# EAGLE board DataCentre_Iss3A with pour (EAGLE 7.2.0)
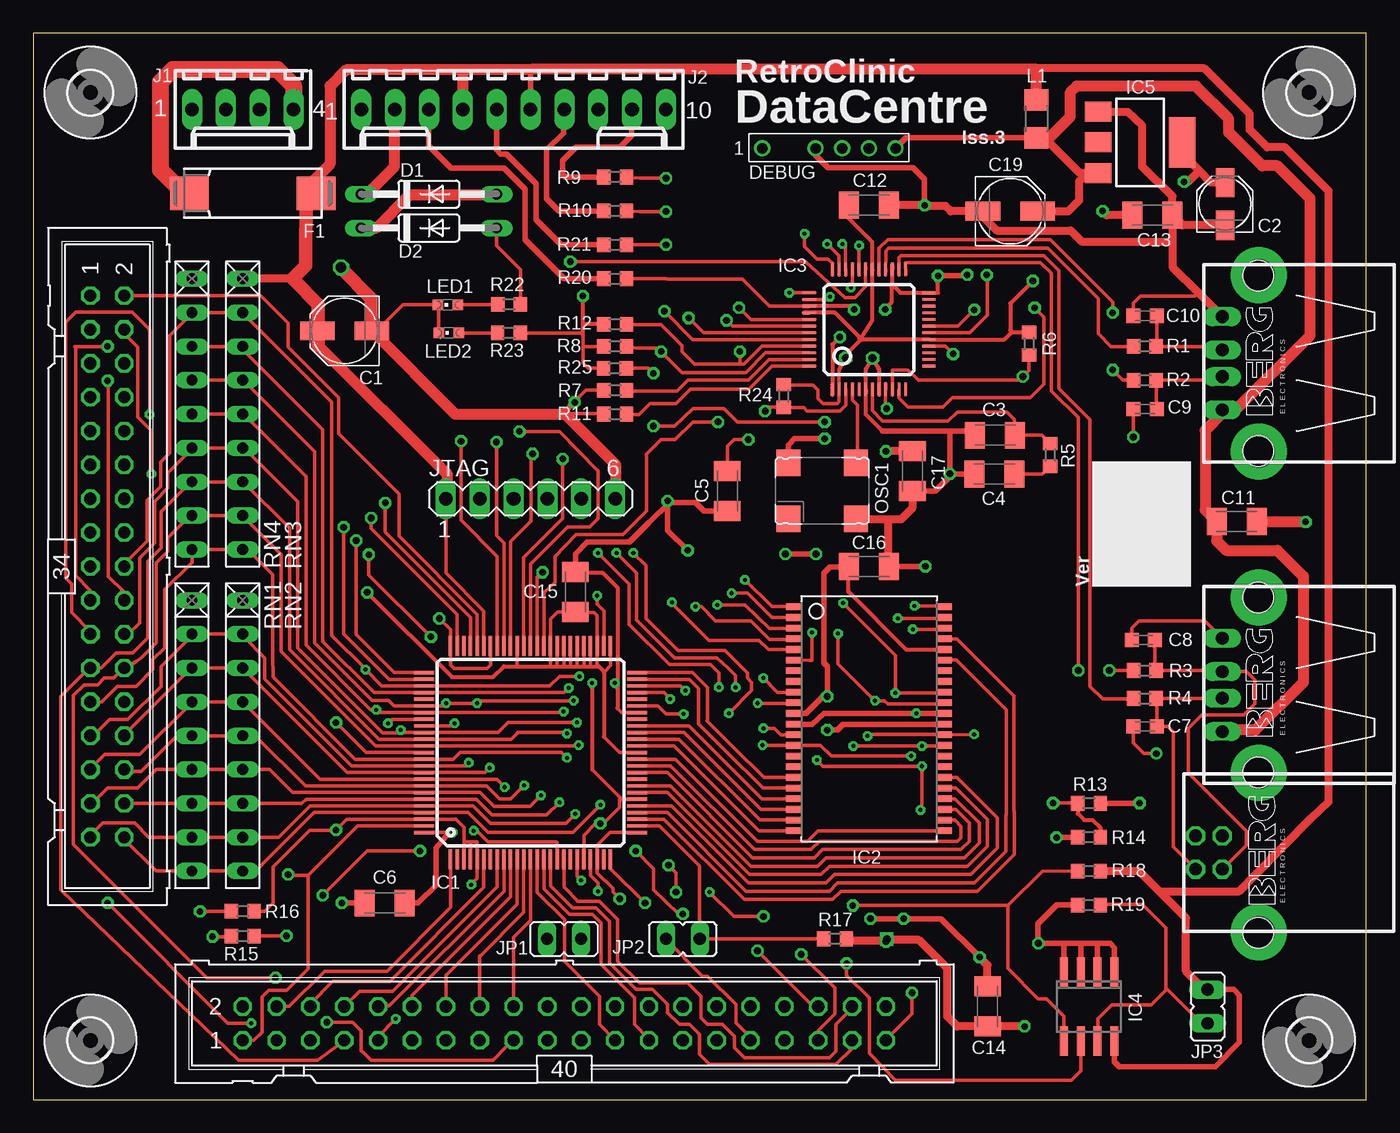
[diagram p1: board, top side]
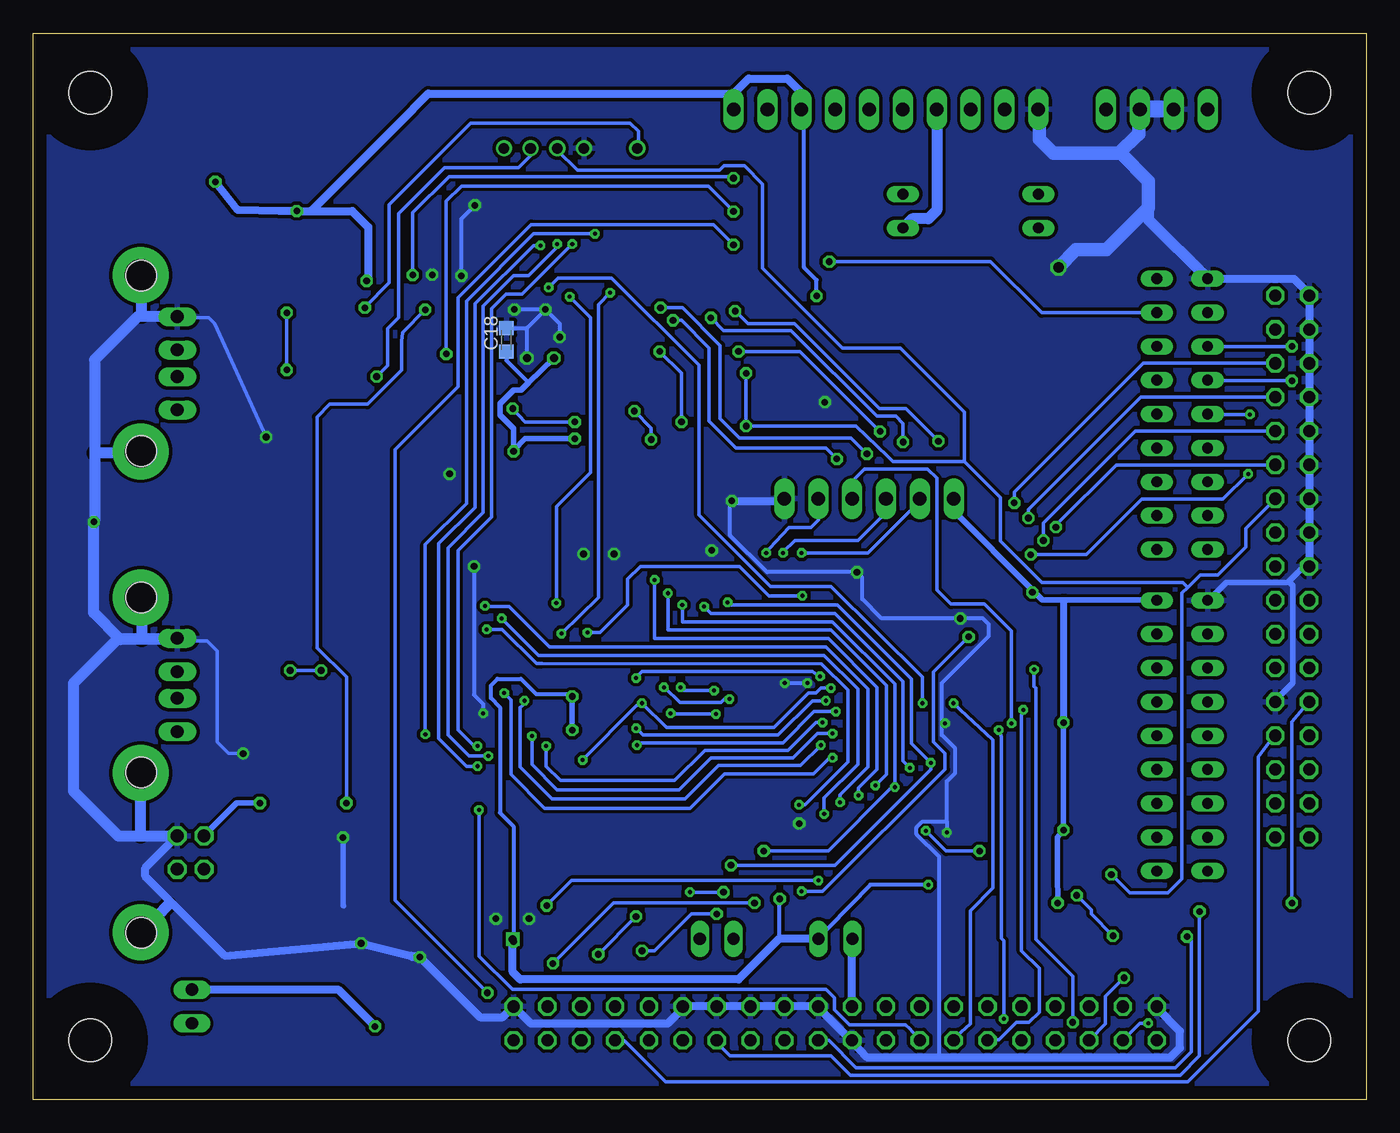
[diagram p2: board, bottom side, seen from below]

Size 100 x 80 mm. Coordinates in mm from the lower left corner, seen from the top.
Outline: 0,0 100,0 100,80 0,80 0,0
Copper layers (1*16): Top 0.035mm / dielectric 1.5mm / Bottom 0.035mm
Design rules "pcb-pool *": minimum track width 6mil, minimum drill 12mil, track to track 6mil, track to pad 6mil, pad to pad 6mil, via to via 6mil, smd to smd 8mil, copper to edge 40mil, drill to drill 20mil, minimum pad ring 8mil, minimum via ring 8mil, stop-mask expansion 3mil, vias tented up to drill 0mil, thermal gap 10mil
Net classes: 0 Signal: width 0.254 mm; 1 Power: width 0.305 mm

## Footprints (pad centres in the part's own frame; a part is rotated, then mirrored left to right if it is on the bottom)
PANASONIC_C = smd 2.6 x 1.4: + 2.05,0; - -2.05,0
PANASONIC_B = smd 2.2 x 1.4: + 1.6,0; - -1.6,0
C1206K = smd 1.5 x 2: 1 -1.5,0; 2 1.5,0
C0603K = smd 1.05 x 1.08: 1 -0.875,0; 2 0.875,0
DO35-10 = drill 0.813 long: A 5.08,0; C -5.08,0
DF3P-06 = drill 0.8: 1 -5,1; 3 -1,1; 4 1,1; 5 3,1; 6 5,1
085CS_1R = smd 2.9 x 2.5: + 4.75,0; - -4.75,0
TQ100 = smd 1.5 x 0.254: 1 -8,6; 2 -8,5.5; 3 -8,5; 4 -8,4.5; 5 -8,4; 6 -8,3.5; 7 -8,3; 8 -8,2.5; 9 -8,2; 10 -8,1.5; 11 -8,1; 12 -8,0.5; 13 -8,0; 14 -8,-0.5; 15 -8,-1; 16 -8,-1.5; 17 -8,-2; 18 -8,-2.5; 19 -8,-3; 20 -8,-3.5; 21 -8,-4; 22 -8,-4.5; 23 -8,-5; 24 -8,-5.5; 25 -8,-6; 51 8,-6; 52 8,-5.5; 53 8,-5; 54 8,-4.5; 55 8,-4; 56 8,-3.5; 57 8,-3; 58 8,-2.5; 59 8,-2; 60 8,-1.5; 61 8,-1; 62 8,-0.5; 63 8,0; 64 8,0.5; 65 8,1; 66 8,1.5; 67 8,2; 68 8,2.5; 69 8,3; 70 8,3.5; 71 8,4; 72 8,4.5; 73 8,5; 74 8,5.5; 75 8,6 | smd 0.254 x 1.5: 26 -6,-8; 27 -5.5,-8; 28 -5,-8; 29 -4.5,-8; 30 -4,-8; 31 -3.5,-8; 32 -3,-8; 33 -2.5,-8; 34 -2,-8; 35 -1.5,-8; 36 -1,-8; 37 -0.5,-8; 38 0,-8; 39 0.5,-8; 40 1,-8; 41 1.5,-8; 42 2,-8; 43 2.5,-8; 44 3,-8; 45 3.5,-8; 46 4,-8; 47 4.5,-8; 48 5,-8; 49 5.5,-8; 50 6,-8; 76 6,8; 77 5.5,8; 78 5,8; 79 4.5,8; 80 4,8; 81 3.5,8; 82 3,8; 83 2.5,8; 84 2,8; 85 1.5,8; 86 1,8; 87 0.5,8; 88 0,8; 89 -0.5,8; 90 -1,8; 91 -1.5,8; 92 -2,8; 93 -2.5,8; 94 -3,8; 95 -3.5,8; 96 -4,8; 97 -4.5,8; 98 -5,8; 99 -5.5,8; 100 -6,8
TSOPII-Z44 = smd 0.5 x 1.2: 1 -8.4,-5.627; 2 -7.6,-5.627; 3 -6.8,-5.627; 4 -6,-5.627; 5 -5.2,-5.627; 6 -4.4,-5.627; 7 -3.6,-5.627; 8 -2.8,-5.627; 9 -2,-5.627; 10 -1.2,-5.627; 11 -0.4,-5.627; 12 0.4,-5.627; 13 1.2,-5.627; 14 2,-5.627; 15 2.8,-5.627; 16 3.6,-5.627; 17 4.4,-5.627; 18 5.2,-5.627; 19 6,-5.627; 20 6.8,-5.627; 21 7.6,-5.627; 22 8.4,-5.627; 23 8.4,5.627; 24 7.6,5.627; 25 6.8,5.627; 26 6,5.627; 27 5.2,5.627; 28 4.4,5.627; 29 3.6,5.627; 30 2.8,5.627; 31 2,5.627; 32 1.2,5.627; 33 0.4,5.627; 34 -0.4,5.627; 35 -1.2,5.627; 36 -2,5.627; 37 -2.8,5.627; 38 -3.6,5.627; 39 -4.4,5.627; 40 -5.2,5.627; 41 -6,5.627; 42 -6.8,5.627; 43 -7.6,5.627; 44 -8.4,5.627
LQFP48 = smd 0.2 x 1: 1 -2.75,-4.5; 2 -2.25,-4.5; 3 -1.75,-4.5; 4 -1.25,-4.5; 5 -0.75,-4.5; 6 -0.25,-4.5; 7 0.25,-4.5; 8 0.75,-4.5; 9 1.25,-4.5; 10 1.75,-4.5; 11 2.25,-4.5; 12 2.75,-4.5; 25 2.75,4.5; 26 2.25,4.5; 27 1.75,4.5; 28 1.25,4.5; 29 0.75,4.5; 30 0.25,4.5; 31 -0.25,4.5; 32 -0.75,4.5; 33 -1.25,4.5; 34 -1.75,4.5; 35 -2.25,4.5; 36 -2.75,4.5 | smd 1 x 0.2: 13 4.5,-2.75; 14 4.5,-2.25; 15 4.5,-1.75; 16 4.5,-1.25; 17 4.5,-0.75; 18 4.5,-0.25; 19 4.5,0.25; 20 4.5,0.75; 21 4.5,1.25; 22 4.5,1.75; 23 4.5,2.25; 24 4.5,2.75; 37 -4.5,2.75; 38 -4.5,2.25; 39 -4.5,1.75; 40 -4.5,1.25; 41 -4.5,0.75; 42 -4.5,0.25; 43 -4.5,-0.25; 44 -4.5,-0.75; 45 -4.5,-1.25; 46 -4.5,-1.75; 47 -4.5,-2.25; 48 -4.5,-2.75
SO-08 = smd 0.6 x 2.2: 1 -1.905,-2.6; 2 -0.635,-2.6; 3 0.635,-2.6; 4 1.905,-2.6; 5 1.905,2.6; 6 0.635,2.6; 7 -0.635,2.6; 8 -1.905,2.6
SOT223 = smd 1.5 x 2: 1 -2.3,-3.15; 2 0,-3.15; 3 2.3,-3.15 | smd 3.8 x 2: 4 0,3.15
ML40 = drill 0.914 octagon: 1 -24.13,-1.27; 2 -24.13,1.27; 3 -21.59,-1.27; 4 -21.59,1.27; 5 -19.05,-1.27; 6 -19.05,1.27; 7 -16.51,-1.27; 8 -16.51,1.27; 9 -13.97,-1.27; 10 -13.97,1.27; 11 -11.43,-1.27; 12 -11.43,1.27; 13 -8.89,-1.27; 14 -8.89,1.27; 15 -6.35,-1.27; 16 -6.35,1.27; 17 -3.81,-1.27; 18 -3.81,1.27; 19 -1.27,-1.27; 20 -1.27,1.27; 21 1.27,-1.27; 22 1.27,1.27; 23 3.81,-1.27; 24 3.81,1.27; 25 6.35,-1.27; 26 6.35,1.27; 27 8.89,-1.27; 28 8.89,1.27; 29 11.43,-1.27; 30 11.43,1.27; 31 13.97,-1.27; 32 13.97,1.27; 33 16.51,-1.27; 34 16.51,1.27; 35 19.05,-1.27; 36 19.05,1.27; 37 21.59,-1.27; 38 21.59,1.27; 39 24.13,-1.27; 40 24.13,1.27
6410-04 = drill 1.016 long: 1 3.81,0; 2 1.27,0; 3 -1.27,0; 4 -3.81,0
6410-10 = drill 1.016 long: 1 11.43,0; 2 8.89,0; 3 6.35,0; 4 3.81,0; 5 1.27,0; 6 -1.27,0; 7 -3.81,0; 8 -6.35,0; 9 -8.89,0; 10 -11.43,0
JP1 = drill 0.914 long: 1 0,-1.27; 2 0,1.27
MA06-1 = drill 1.016 long: 1 -6.35,0; 2 -3.81,0; 3 -1.27,0; 4 1.27,0; 5 3.81,0; 6 6.35,0
R1206 = smd 1.6 x 1.803: 1 -1.422,0; 2 1.422,0
CHIPLED_0603 = smd 0.8 x 0.8: A 0,-0.75; C 0,0.75
XTAL-CSX750 = smd 1.8 x 2: 1 -2.54,-2.1; 2 2.54,-2.1; 3 2.54,2.1; 4 -2.54,2.1
ML34 = drill 0.914 octagon: 1 -20.32,-1.27; 2 -20.32,1.27; 3 -17.78,-1.27; 4 -17.78,1.27; 5 -15.24,-1.27; 6 -15.24,1.27; 7 -12.7,-1.27; 8 -12.7,1.27; 9 -10.16,-1.27; 10 -10.16,1.27; 11 -7.62,-1.27; 12 -7.62,1.27; 13 -5.08,-1.27; 14 -5.08,1.27; 15 -2.54,-1.27; 16 -2.54,1.27; 17 0,-1.27; 18 0,1.27; 19 2.54,-1.27; 20 2.54,1.27; 21 5.08,-1.27; 22 5.08,1.27; 23 7.62,-1.27; 24 7.62,1.27; 25 10.16,-1.27; 26 10.16,1.27; 27 12.7,-1.27; 28 12.7,1.27; 29 15.24,-1.27; 30 15.24,1.27; 31 17.78,-1.27; 32 17.78,1.27; 33 20.32,-1.27; 34 20.32,1.27
R0603 = smd 1 x 1.1: 1 -0.85,0; 2 0.85,0
RN-9 = drill 0.813 long: 1 -10.16,0; 2 -7.62,0; 3 -5.08,0; 4 -2.54,0; 5 0,0; 6 2.54,0; 7 5.08,0; 8 7.62,0; 9 10.16,0
3,2 = hole 3.2: 0,0
PN87520 = drill 0.95 long: 1 -3.5,2.71; 2 -1,2.71; 3 1,2.71; 4 3.5,2.71 | hole 2.3: -6.57,0; 6.57,0
PN61729 = drill 0.95 octagon: 1 1.25,4.71; 2 -1.25,4.71; 3 -1.25,2.71; 4 1.25,2.71 | hole 2.3: -6.02,0; 6.02,0

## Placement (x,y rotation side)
C1  47uF  [PANASONIC_C]  23.36,57.68 180 top
C2  22uF  [PANASONIC_B]  89.4,67.19 90 top
C3  1nF  [C1206K]  72.16,49.85 0 top
C4  10nF  [C1206K]  72.1,46.94 180 top
C5  100nF  [C1206K]  52.07,45.68 270 top
C6  100nF  [C1206K]  26.36,14.74 0 top
C7  47pF  [C0603K]  83.41,27.99 0 top
C8  47pF  [C0603K]  83.28,34.48 0 top
C9  47pF  [C0603K]  83.41,51.81 0 top
C10  47pF  [C0603K]  83.41,58.8 0 top
C11  100nF  [C1206K]  90.28,43.37 0 top
C12  100nF  [C1206K]  62.7,67.11 0 top
C13  100nF  [C1206K]  83.97,66.35 0 top
C14  100nF  [C1206K]  71.59,6.98 90 top
C15  100nF  [C1206K]  40.67,38.09 90 top
C16  100nF  [C1206K]  62.7,40 0 top
C17  100nF  [C1206K]  65.95,47.16 270 top
C18  100nF  [C0603K]  64.51,57.01 90 bottom
C19  47uF  [PANASONIC_C]  73.3,66.65 0 top
D1  1N4001  [DO35-10]  29.68,67.94 0 top
D2  1N4001  [DO35-10]  29.68,65.4 0 top
DEBUG  [DF3P-06]  59.69,70.37 0 top
F1  [085CS_1R]  16.47,68 180 top
IC1  XC9572TQ100  [TQ100]  37.3,26.03 90 top
IC2  62LV8001  [TSOPII-Z44]  62.7,28.57 270 top
IC3  VNC1L-1A  [LQFP48]  62.7,57.78 0 top
IC4  24LC512  [SO-08]  79.21,6.98 180 top
IC5  TS1117BCW33  [SOT223]  83.05,71.82 270 top
IDE  IDE  [ML40]  39.84,5.71 0 top
J1  22-27-2041-04  [6410-04]  15.71,74.29 180 top
J2  22-27-2101-10  [6410-10]  36.03,74.29 180 top
JP1  IDEPWR  [JP1]  39.82,12.06 90 top
JP2  SEL  [JP1]  48.73,12.06 90 top
JP3  WPROT  [JP1]  88.1,6.98 0 top
JTAG  [MA06-1]  37.3,45.08 0 top
L1  600R  [R1206]  75.25,73.58 90 top
LED1  [CHIPLED_0603]  31.11,59.63 90 top
LED2  [CHIPLED_0603]  31.17,57.52 90 top
OSC1  [XTAL-CSX750]  59.19,45.68 0 top
PL1  1MHZ  [ML34]  5.55,40 270 top
R1  27R  [R0603]  83.39,56.51 0 top
R2  27R  [R0603]  83.39,53.97 0 top
R3  27R  [R0603]  83.39,32.19 0 top
R4  27R  [R0603]  83.39,30.09 0 top
R5  180R  [R0603]  76.29,48.37 90 top
R6  47K  [R0603]  74.71,56.71 90 top
R7  47K  [R0603]  43.65,53.21 0 top
R8  47K  [R0603]  43.65,56.51 0 top
R9  330R  [R0603]  43.65,69.21 0 top
R10  330R  [R0603]  43.65,66.67 0 top
R11  10K  [R0603]  43.65,51.43 180 top
R12  47K  [R0603]  43.65,58.17 180 top
R13  100K  [R0603]  79.21,22.22 0 top
R14  100K  [R0603]  79.21,19.68 0 top
R15  1k  [R0603]  15.72,12.26 180 top
R16  4k7  [R0603]  15.72,14.13 180 top
R17  4k7  [R0603]  60.16,12.06 0 top
R18  4k7  [R0603]  79.21,17.14 0 top
R19  4k7  [R0603]  79.21,14.6 0 top
R20  470R  [R0603]  43.65,61.59 180 top
R21  470R  [R0603]  43.65,64.13 0 top
R22  470R  [R0603]  35.7,59.66 180 top
R23  330R  [R0603]  35.69,57.52 180 top
R24  0R  [R0603]  56.29,52.79 270 top
R25  47K  [R0603]  43.62,54.87 0 top
RN1  2k2  [RN-9]  11.9,27.3 270 top
RN2  2k2  [RN-9]  15.71,27.3 270 top
RN3  2k2  [RN-9]  15.71,51.43 270 top
RN4  2k2  [RN-9]  11.9,51.43 270 top
U$1  [3,2]  95.72,75.56 0 top
U$2  [3,2]  95.72,4.44 0 top
U$3  [3,2]  4.28,4.44 0 top
U$4  [3,2]  4.28,75.56 0 top
X1  USB2  [PN87520]  91.91,55.24 90 top
X2  USB1A  [PN87520]  91.91,31.11 90 top
X3  USB1B  [PN61729]  91.91,18.54 90 top

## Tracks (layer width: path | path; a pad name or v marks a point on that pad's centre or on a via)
!ACT  (via drill 0.5)
  Top 0.254: v65.93,8 65.93,6.43 63.97,4.47 IDE.39 | v47.47,64.13 R21.2
  Bottom 0.254: v65.93,8 72.86,14.93 72.86,48.76 68.13,53.49 68.13,60.16 62.65,65.65 48.98,65.65 48.97,65.63 v47.47,64.13
!DACK  (via drill 0.5)
  Top 0.254: 42.37,47.13 42.37,43.6 41.73,42.97 40.1,42.97 37.3,40.17 IC1.63 | 42.37,47.13 42.37,47.19 | IC3.46 54.92,56.03 53.45,54.56 48.66,54.56 47.03,56.19 | 47.03,56.19 46.84,56.39 45.27,56.39 R8.2 | v47.1,56.13 46.97,56.13 47.03,56.19 | v36.47,50.13 39.47,50.13 42.34,47.19 42.37,47.13
  Bottom 0.254: v47.1,56.13 42.47,56.13 v36.47,50.13
!DREQ  (via drill 0.5)
  Top 0: IC3.45 58.22,56.51 58.22,56.53
  Top 0.254: 58.64,56.53 58.22,56.53 54.67,56.53 53.33,55.19 53.14,55.19 | 58.64,56.53 IC3.45 | 53.14,55.19 49.61,55.19 48.66,56.13 48.66,56.57 47.09,58.15 44.52,58.15 R12.1 | v51.37,50.84 49.48,50.84 48.16,49.52 47.09,49.52 46.02,48.45 46.02,44.16 44.25,42.4 40.73,42.4 39.15,40.76 39.15,38.81 38.33,38.05 38.3,38.02 IC1.61 | v53.01,56.13 53.01,55.31 53.14,55.19
  Bottom 0.254: v51.37,50.84 51.37,54.5 v53.01,56.13
!IDECS0
  Top 0.254: IDE.37 61.41,3.81 60.22,2.63 50.72,2.63 49.97,3.38 49.97,4.88 49.22,5.63 48.47,5.63 47.59,6.5 47.59,7.13 46.47,8.26 45.22,8.26 43.22,10.26 43.22,13.38 42.22,14.38 40.47,14.38 38.8,16.05 IC1.16
!IDECS1
  Top 0.254: IDE.38 61.43,6.84 60.22,5.63 60.22,3.63 59.72,3.13 53.34,3.13 52.59,3.88 52.59,4.75 51.72,5.63 50.59,5.63 50.09,6.13 50.09,7.75 49.09,8.76 45.47,8.76 43.84,10.38 43.84,13.51 42.47,14.88 40.89,14.88 | 40.84,14.88 40.89,14.88 | IC1.18 39.8,15.97 40.89,14.88
!IDEINT
  Top 0.254: IDE.31 53.81,4.67 52.72,5.75 52.72,7.13 50.59,9.26 50.22,9.26 47.41,12.06 | 47.41,12.06 47.34,12.13 | 47.41,12.06 JP2.2
!IDEINTA
  Top 0.254: R17.1 JP2.1 49.98,12.08 49.98,17.52 46.97,20.53 IC1.27
!IDERD
  Top 0.254: IDE.25 46.19,4.54 45.09,5.63 45.09,7.63 42.59,10.13 42.59,13.26 41.97,13.88 40.22,13.88 38.3,15.8 IC1.15
!IDEWR
  Top 0.254: IDE.23 42.47,5.63 42.47,7.75 39.84,10.38 39.84,13.51 37.8,15.55 IC1.14
!IRQ  (via drill 0.5 pad 0.25)
  Top 0.254: 31.81,33.97 IC1.74 31.8,36.4 25.36,42.84 25.36,43.63 v25.34,43.64
  Bottom 0.254: PL1.8 16.9,52.7 25.34,44.26 v25.34,43.64
!NMI  (via drill 0.5 pad 0.25)
  Top 0.254: v26.41,44.76 26.41,42.57 32.8,36.18 IC1.72
  Bottom 0.254: PL1.6 16.73,55.24 26.41,45.57 v26.41,44.76
!PGFC  (via drill 0.5 pad 0.25)
  Top 0.254: v24.22,41.94 24.22,34.88 27.07,32.03 IC1.76
  Bottom 0.254: PL1.10 17.31,50.16 24.22,43.26 v24.22,41.94
!PGFD  (via drill 0.5 pad 0.25)
  Top 0.254: v23.28,42.94 23.28,34.94 26.7,31.53 IC1.77
  Bottom 0.254: PL1.12 18.73,47.62 23.28,43.09 23.28,42.82 v23.28,42.94
!RCE  (via drill 0.3)
  Top 0.254: v58.43,35.03 58.43,32.95 58.24,32.95 IC2.6 | v42.3,37.8 42.3,37.17 42.81,36.67 42.81,34.78 IC1.52
  Bottom 0.254: v58.43,35.03 57.48,35.03 55.41,37.11 55.41,39.06 54.46,40.01 47.03,40.01 44.82,37.8 v42.3,37.8
!ROE
  Top 0.254: IC2.41 69.28,34.57 73.55,30.29 73.55,21.67 73.59,21.63 73.59,18.38 70.84,15.63 60.59,15.63 59.97,15.01 53.34,15.01 47.32,21.03 IC1.28 45.24,21.03
!RST  (via drill 0.5)
  Top 0.254: IDE.1 16.53,4.43 17.16,5.06 17.16,7.7 17.67,8.19 18.99,8.19 20.6,9.8 20.6,16.81 | 29.32,20.53 IC1.99 24.32,20.53 20.6,16.81 | v64.04,51.85 63.95,51.96 63.95,53.72 IC3.9 | v46.52,50.53 48.1,50.53 49.48,51.85 51.81,51.85 52.82,50.84 v59.38,50.84 | R25.2 46.14,54.87 v46.52,54.5 | 20.6,16.81 19.19,16.81 v19.12,16.88
  Bottom 0.254: PL1.14 7.32,44.55 9.04,42.84 9.04,41.45 11.12,39.38 12.44,39.38 13.38,38.43 | 13.38,38.43 13.83,37.99 13.83,16.57 14.9,15.5 17.73,15.5 v19.12,16.88 | 30.14,47.88 35.5,47.88 35.88,48.26 38.27,50.53 v46.52,50.53 v46.52,54.5 | 30.14,47.88 27.43,45.17 27.43,41.9 24.35,38.81 13.76,38.81 13.38,38.43 | DEBUG.4 60.69,71.24 59.17,69.72 48.52,69.72 48.19,70.06 46.65,70.06 45.29,68.66 45.29,62.4 39.28,56.39 34.93,56.39 30.14,51.6 30.14,47.88 | v59.38,50.84 63.09,50.84 v64.04,51.85
!RWE
  Top 0.254: IC2.17 54.8,24.17 52.51,26.46 50.56,28.41 50.57,28.42 50.57,30.92 49.46,32.03 IC1.50 45.24,32.03
AD0  (via drill 0.3, 0.5)
  Top 0.254: RN1.2 11.88,34.92 11.85,34.88 | RN1.2 RN2.2 15.71,34.77 15.73,34.77 17.35,33.14 17.35,31.56 23.89,25.03 IC1.90 32.43,25.03 v32.66,25.26 | RN1.2 11.9,34.81 9.6,32.51 9.6,31 7.09,28.5 5.72,28.5 4.34,27.13 4.28,27.2 PL1.27 | v47.91,37.3 47.91,37.23 50.68,34.46 54.46,34.46 55.15,33.77 57.11,33.77 57.1,33.77 IC2.5 | v50.74,15.56 52.57,13.73 v54.78,13.73 | v47.66,17.58 48.22,17.01 v48.22,15.56 | IDE.35 58.87,5.17 60.13,6.43 60.13,8.38 v57.61,10.9
  Bottom 0.254: v47.91,37.3 47.72,37.11 39.66,37.11 34.11,31.56 34.11,26.71 v32.66,25.26 32.66,24.76 39.84,17.58 v47.66,17.58 | v48.22,15.56 v50.74,15.56 | v57.61,10.9 v54.78,13.73
AD1  (via drill 0.3)
  Top 0.254: RN2.3 | 11.9,32.45 11.85,32.51 | 11.9,32.45 RN1.3 11.85,32.38 6.82,27.36 PL1.28 | RN2.3 11.97,32.38 11.9,32.45 | v49.67,36.98 50.11,36.98 51.19,35.91 53.83,35.91 55.22,34.52 57.11,34.52 57.07,34.56 IC2.4 | RN2.3 23.56,24.53 IC1.91 33.88,24.53 v34.24,24.88
  Bottom 0.254: v34.24,24.88 34.74,25.39 34.74,31.37 39.84,36.48 49.17,36.48 v49.67,36.98 | IDE.33 55.97,4.41 55.66,4.41 52.57,1.32 13.38,1.32 8.09,6.62 8.09,25.7 7.34,26.71 PL1.28
AD2  (via drill 0.3, 0.5)
  Top 0.254: RN2.4 15.76,29.84 | RN1.4 11.68,29.84 11.6,29.75 | RN1.4 RN2.4 | RN1.4 11.9,29.81 7.97,25.88 5.34,25.88 4.28,24.81 PL1.29 | v51.31,37.11 53.39,37.11 55.22,35.34 57.17,35.34 57.14,35.37 IC2.3 | v54.34,11.15 58.24,7.25 IDE.36 | v45.2,18.65 46.52,17.32 46.52,15.75 48.41,13.92 v48.73,13.92 | v35.37,23.44 34.78,24.03 IC1.92 21.52,24.03 RN2.4
  Bottom 0.254: v51.31,37.11 51.31,35.85 40.03,35.85 35.37,31.18 v35.37,23.44 35.62,23.44 40.35,18.65 v45.2,18.65 | v54.34,11.15 53.39,11.15 50.62,13.92 v48.73,13.92
AD3  (via drill 0.3)
  Top 0.254: RN1.5 11.85,27.25 | RN1.5 RN2.5 15.75,27.26 16.7,27.26 20.43,23.53 IC1.93 34.02,23.53 35,22.55 35.81,22.55 v36.82,23.56 | RN1.5 10.77,27.3 8.1,24.63 6.97,24.63 6.84,24.76 PL1.30 | v52.38,37.99 53.58,37.99 55.41,36.16 57.04,36.16 57.05,36.17 IC2.2
  Bottom 0.254: v36.82,23.56 36,24.38 36,31.06 40.16,35.22 52.38,35.22 v52.38,37.99
AD4  (via drill 0.3)
  Top 0.254: RN1.6 11.73,24.76 11.72,24.75 | RN1.6 RN2.6 17.71,24.76 19.45,23.03 IC1.94 33.51,23.03 34.55,21.99 37.26,21.99 v38.08,22.81 | RN1.6 9.23,24.76 7.84,23.38 5.59,23.38 4.34,22.13 4.28,22.2 PL1.31 | v53.39,39 55.41,36.98 57.04,36.98 57.05,36.97 IC2.1
  Bottom 0.254: v38.08,22.81 38.08,23.37 36.7,24.76 36.7,30.93 40.35,34.59 53.39,34.59 v53.39,39
AD5  (via drill 0.3)
  Top 0.254: 15.71,22.24 15.72,22.25 | 15.71,22.24 RN2.7 20.14,22.22 20.45,22.53 IC1.95 33.25,22.53 34.43,21.36 38.52,21.36 v39.47,22.3 | 15.71,22.24 15.69,22.22 RN1.7 PL1.32 6.75,22.22 6.72,22.25 | IC2.44 68.33,36.99 68.38,37.04 v66.12,37.04
  Bottom 0.254: v39.47,22.3 39.47,22.87 37.39,24.95 37.39,30.81 40.54,33.96 61.27,33.96 64.29,36.98 66.05,36.98 v66.12,37.04
AD6  (via drill 0.3)
  Top 0.254: RN1.8 11.77,19.68 11.72,19.63 | RN1.8 RN2.8 18.42,19.68 20.77,22.03 IC1.96 33,22.03 34.3,20.73 39.97,20.73 v40.66,21.42 | RN1.8 8.67,19.68 7.59,20.75 5.22,20.75 4.22,19.75 4.28,19.7 PL1.33 | IC2.43 68.33,36.22 68.32,36.23 68.19,36.1 v64.86,36.1
  Bottom 0.254: v40.66,21.42 40.66,22.62 38.14,25.14 38.14,30.81 40.66,33.33 62.08,33.33 v64.86,36.1
AD7  (via drill 0.3)
  Top 0.254: 29.32,21.53 IC1.97 | 11.97,17.14 RN1.9 9.21,17.14 6.72,19.63 6.77,19.68 PL1.34 | 11.97,17.14 RN2.9 16.69,17.14 21.08,21.53 IC1.97 | 11.97,17.14 11.97,17 | v42.55,22.11 40.48,20.03 34.11,20.03 32.62,21.53 IC1.97 | IC2.42 68.36,35.37 68.38,35.34 68.32,35.28 v65.99,35.28
  Bottom 0.254: v42.55,22.11 42.11,22.11 38.9,25.33 38.9,30.74 40.85,32.7 61.82,32.73 | 61.82,32.73 61.91,32.73 | v65.99,35.28 64.83,35.28 62.23,32.73 61.87,32.73 61.82,32.73
ADR8
  Top 0.254: IC2.39 69.25,32.97 72.99,29.23 72.99,21.36 72.97,21.38 72.97,18.63 70.59,16.25 60.34,16.25 59.72,15.63 53.47,15.63 47.57,21.53 IC1.29
ADR9
  Top 0.254: IC2.28 69.3,24.17 72.34,21.13 72.34,18.88 70.34,16.88 60.09,16.88 59.47,16.25 53.65,16.25 47.88,22.03 IC1.30
ADR10
  Top 0.254: IC2.27 69.23,23.37 71.59,21 71.59,19 70.09,17.5 59.72,17.5 59.09,16.88 53.72,16.88 47.57,23.03 IC1.32
ADR11
  Top 0.254: IC2.26 69.16,22.57 70.97,20.75 70.97,19.25 69.84,18.13 59.47,18.13 58.84,17.5 53.84,17.5 47.82,23.53 IC1.33
ADR12
  Top 0.254: IC2.25 69.2,21.77 70.22,20.75 70.22,19.38 69.59,18.75 59.22,18.75 58.59,18.13 53.97,18.13 47.57,24.53 IC1.35
ADR13
  Top 0.254: IC2.24 69.13,20.97 69.59,20.5 69.59,19.63 69.34,19.38 58.97,19.38 58.34,18.75 54.09,18.75 47.82,25.03 IC1.36 45.24,25.03
ADR14
  Top 0.254: IC2.23 58.88,20.17 58.09,19.38 54.34,19.38 48.2,25.53 IC1.37
ADR15
  Top 0.254: IC2.22 54.43,20.17 48.07,26.53 IC1.39
ADR16
  Top 0.254: IC2.21 54.5,20.97 48.45,27.03 IC1.40 45.24,27.03
ADR17
  Top 0.254: IC2.20 54.58,21.77 48.82,27.53 IC1.41
ADR18
  Top 0.254: IC2.19 54.66,22.57 49.2,28.03 IC1.42
ADR19
  Top 0.254: IC2.18 54.73,23.37 52,26.08 49.91,28.18 49.91,30.86 49.23,31.53 IC1.49
DB0  (via drill 0.3, 0.5)
  Top 0.254: 15.71,59.02 22.4,52.33 22.4,34.81 24.91,32.29 v24.91,32.26 26.14,31.03 IC1.78 38.74,31.03 39.47,31.75 v40.98,31.75 | 15.71,59.02 RN3.2 | RN4.2 15.68,59.05 15.71,59.02 | RN4.2 12.08,59.05 12.19,59.16 | PL1.18 6.82,40.18 8.53,41.9 8.53,44.98 9.54,45.99 9.54,47.82 10.24,48.51 10.24,57.33 11.96,59.05 | 11.96,59.05 12,59.09 | RN4.2 11.96,59.05 | IC2.9 57.06,30.57 57.04,30.55 55.85,30.55 v54.78,31.63 | v40.29,62.87 57.93,62.87 60.89,60.16 61.64,60.16 62.44,60.98 62.44,62.71 IC3.31 | v22.02,5.8 23.97,5.8 24.6,5.17 24.6,3.65 24.72,3.53 25.36,2.96 34.49,2.96 35.56,4.03 IDE.17
  Bottom 0.254: v40.98,31.75 41.04,31.75 41.55,32.13 54.34,32.13 v54.78,31.63 | v40.29,62.87 28.19,62.87 24.35,59.03 17.48,59.03 RN3.2 | v24.91,32.26 24.91,31 24.79,30.87 24.79,12.03 22.02,9.26 v22.02,5.8
DB1  (via drill 0.3, 0.5)
  Top 0.254: 15.71,56.39 15.72,56.38 | 15.71,56.39 RN3.3 15.71,56.27 21.72,50.26 21.72,34.38 25.57,30.53 IC1.79 39.82,30.53 v40.16,30.87 | RN4.3 15.59,56.51 15.71,56.39 | PL1.19 4.28,38.21 3.18,39.31 3.18,56.45 3.12,56.51 v5.57,56.51 | IC2.10 57.04,29.74 v54.34,29.74 | v61.96,64.07 61.95,61.85 IC3.32 | v58.78,25.47 59.24,25.01 v66.68,25.01 66.68,22.19 v66.57,21.72
  Bottom 0.254: 11.9,56.42 11.94,56.39 | RN4.3 11.9,56.42 | v5.57,56.51 11.81,56.51 11.9,56.42 | v40.16,30.87 40.92,30.87 41.29,30.49 41.86,30.49 44.44,27.91 52.51,27.91 v54.34,29.74 54.78,29.55 v58.78,25.47 | v61.96,64.07 62.46,64.07 66.87,59.72 66.87,44.41 69.58,41.71 69.58,27.09 67.5,25.01 v66.68,25.01 67.06,25.01 | IDE.15 33.86,4.85 34.24,5.29 34.55,5.61 38.77,5.61 39.91,6.74 39.91,7.62 40.54,8.25 64.04,8.25 66.57,10.75 v66.57,21.72
DB2  (via drill 0.3, 0.5)
  Top 0.254: 15.71,53.89 15.72,53.88 | 15.71,53.89 RN3.4 15.76,53.97 21.09,48.63 21.09,34.26 25.42,29.93 26.66,29.93 27.07,29.53 IC1.81 | RN4.4 15.63,53.97 15.71,53.89 | 29.24,29.53 IC1.81 | PL1.20 6.82,38.07 5.64,39.25 5.64,53.87 v5.57,53.93 | v54.78,27.85 55.59,27.85 56.1,27.34 56.98,27.34 57.04,27.4 IC2.13 | v61.33,60.92 61.45,61.05 61.45,62.71 IC3.33 | IC1.81 30.76,29.53 v30.96,29.74 v33.29,29.74 33.48,29.93 v40.54,29.93
  Bottom 0.254: 12.04,53.97 12.06,53.99 | RN4.4 12.04,53.97 | v5.57,53.93 12,53.93 12.04,53.97 | v40.54,29.93 41.55,29.93 44.13,27.34 54.27,27.34 v54.78,27.85 | v61.33,60.92 60.63,61.61 56.6,61.61 50.05,55.12 50.05,43.85 44.7,38.49 40.16,38.49 33.29,31.69 v33.29,29.74 | v30.96,29.74 28,26.96 28,15.88 29.7,14.18 29.7,5.67 30.39,5.04 IDE.13
DB3  (via drill 0.3)
  Top 0: IC3.34 60.97,62.38 60.95,62.38
  Top 0.254: RN4.5 RN3.5 15.79,51.43 20.47,46.76 20.47,34.09 25.31,29.25 25.72,29.25 v25.73,29.23 25.93,29.03 IC1.82 | 29.24,29.03 IC1.82 | PL1.21 4.28,35.12 2.86,36.54 2.86,38.68 2.42,39.12 2.42,58.34 3.18,59.09 7.4,59.09 8.72,57.77 v8.72,51.41 | v54.71,26.59 56.92,26.59 56.98,26.52 57.03,26.57 IC2.14 59.06,26.59 59.88,25.77 v65.86,25.77 | v60.7,64.2 60.94,63.96 60.95,62.38 60.95,61.86 | 60.95,61.86 IC3.34 | IC1.82 39.71,29.03 v39.78,29.11
  Bottom 0.254: 12,51.41 11.98,51.43 RN4.5 | 12,51.41 v8.72,51.41 | 12,51.41 12.06,51.35 | v39.78,29.11 41.42,29.11 43.75,26.77 54.52,26.77 v54.71,26.59 | v60.7,64.2 60.7,63.95 62.84,61.8 63.97,61.8 66.24,59.54 66.24,44.04 68.89,41.39 68.89,27.34 67.31,25.77 v65.86,25.77 | IDE.11 28.38,4.47 27.56,4.47 26.24,5.8 25.29,5.8 24.54,6.55 24.54,9.83 25.86,11.15 25.86,28.85 25.8,28.92 v25.73,29.23
DB4  (via drill 0.3)
  Top 0: IC3.35 60.47,62.38 60.45,62.38
  Top 0.254: RN3.6 15.84,48.89 19.84,44.88 19.84,33.88 26.22,27.5 27.34,27.5 v27.56,27.72 27.75,27.53 IC1.85 34.87,27.53 35.62,28.29 v40.79,28.29 | PL1.22 7.13,34.92 7.97,35.76 7.97,40.63 9.1,41.76 9.1,44.88 10.1,45.88 10.1,47.01 11.97,48.88 11.96,48.89 | 11.96,48.89 RN4.6 | RN3.6 11.96,48.89 | RN3.6 15.85,48.76 | IC2.31 68.32,26.59 68.26,26.52 v66.68,26.52 v61.52,26.52 | v59.56,64.2 60.45,63.32 60.45,62.38 60.45,61.86 | 60.45,61.86 IC3.35 | v27.18,6.05 25.86,4.72 IDE.9
  Bottom 0.254: v40.79,28.29 41.29,28.29 43.37,26.21 49.61,26.21 51.88,23.94 60.45,23.94 61.52,25.01 v61.52,26.52 | v59.56,64.2 63.34,60.42 64.54,60.42 65.61,59.35 65.61,43.72 68.13,41.2 68.13,27.72 66.94,26.52 v66.68,26.52 | v27.18,6.05 27.18,11.91 27.37,12.1 27.37,27.22 v27.56,27.72
DB5  (via drill 0.3)
  Top 0: IC3.36 59.97,62.63 59.95,62.75
  Top 0.254: 11.9,46.31 11.85,46.26 | 11.9,46.31 RN4.7 11.88,46.35 11.85,46.38 9.6,44.13 9.6,41.38 8.6,40.38 8.6,34.63 7.47,33.51 6.22,33.51 5.09,32.38 PL1.23 3.62,31.81 2.04,30.24 2.04,15.75 15.4,2.96 21.32,2.96 22.9,4.09 23.4,4.54 IDE.7 | 11.9,46.31 11.94,46.35 RN3.7 15.75,46.35 19.22,42.88 19.22,33.76 25.95,27.03 IC1.86 35.86,27.03 36.36,27.53 | 36.32,27.53 36.36,27.53 | 36.36,27.53 39.97,27.53 v40.03,27.47 | v62.59,27.28 62.97,27.4 68.32,27.4 68.33,27.4 IC2.32 70.34,27.4 v70.59,27.4 | v57.86,64.95 57.86,64.01 58.81,63.06 59.63,63.06 59.95,62.75 59.95,62.38 59.95,61.86 | 59.95,61.86 IC3.36
  Bottom 0.254: v40.03,27.47 41.17,27.47 42.99,25.64 49.17,25.64 51.56,23.25 60.7,23.25 62.59,25.14 v62.59,27.28 | v57.86,64.95 62.46,64.95 67.5,59.91 67.5,44.73 70.59,41.64 v70.59,27.4
DB6  (via drill 0.3, 0.5)
  Top 0.254: 11.9,43.83 11.85,43.88 | 11.9,43.83 RN4.8 11.78,43.81 10.1,42.13 10.1,41.13 9.22,40.26 9.22,34.26 8.1,33.13 7.72,32.88 6.97,32.38 PL1.24 6.01,31.63 5.32,31.63 4.82,31.12 3.81,31.12 2.99,30.3 2.99,19.15 13.01,9.14 v18.17,9.14 | 11.9,43.83 11.92,43.81 RN3.8 15.71,43.77 18.59,40.88 18.59,33.63 25.7,26.53 IC1.87 40.86,26.53 v40.92,26.59 | IC2.35 68.33,29.86 68.32,29.86 68.13,29.67 64.1,29.67 63.85,29.93 v63.16,29.93 60.38,32.7 v60.38,34.97 | v56.73,60.54 56.79,60.53 58.63,60.53 IC3.37
  Bottom 0.254: v40.92,26.59 42.43,25.07 48.6,25.07 51.12,22.55 61.08,22.55 63.47,24.95 63.47,29.42 63.16,29.67 v63.16,29.93 | v56.73,60.54 57.61,59.66 57.61,37.67 v60.38,34.97 | v18.17,9.14 19.56,7.75 19.56,5.67 20.69,4.54 IDE.5
DB7  (via drill 0.3, 0.5)
  Top 0: IC3.38 58.22,60.01 58.22,60.03
  Top 0.254: RN3.9 16.08,41.27 17.97,39.38 17.97,33.38 17.98,31.69 24.14,25.53 IC1.89 31.49,25.53 32,26.04 39.63,26.04 v40.03,25.64 | RN3.9 15.83,41.27 15.85,41.26 | RN3.9 RN4.9 11.9,40.31 9.85,38.26 9.85,33.88 8.97,33.01 8.97,32.26 7.72,31 6.29,31 5.12,29.84 PL1.25 | IC2.36 68.37,30.57 68.38,30.55 68.32,30.49 v64.67,30.49 64.67,33.3 v60.76,37.24 | v59.75,60.23 59.56,60.03 58.22,60.03 57.77,60.03 | 57.77,60.03 IC3.38 | v16.35,5.73 14.58,5.73 v5.57,14.74
  Bottom 0.254: v40.03,25.64 40.29,25.64 41.48,24.44 48.16,24.44 50.74,21.86 61.64,21.86 64.16,24.38 64.16,29.99 v64.67,30.49 | v60.76,37.24 60.76,44.48 58.18,47.06 58.18,58.65 v59.75,60.23 | v16.35,5.73 16.98,5.73 IDE.3 | v5.57,14.74 5.57,28.35 4.75,29.29 PL1.25
DRQ  (via drill 0.5)
  Top 0.254: v13.45,12.22 14.84,12.22 R15.2
  Bottom 0.254: IDE.21 40.32,4.44 38.27,2.39 14.33,2.39 13.13,3.59 13.13,11.91 v13.45,12.22
DRQA  (via drill 0.3, 0.5)
  Top 0.254: v33.04,20.16 33.29,20.16 34.11,19.34 38.84,19.34 39.23,19.34 39.3,19.28 IC1.17 | v29.01,18.65 25.04,18.65 v21.72,15.32 | v18.99,12.29 16.6,12.29 R15.1
  Bottom 0.254: v29.01,18.65 31.53,18.65 v33.04,20.16 | v21.72,15.32 20.63,14.24 20.63,13.92 v18.99,12.29
GND  (via drill 0.3, 0.5, 0.6, 0.8)
  Top 0: IC3.1 59.97,53.63 59.95,53.63 | 62.46,52.98 62.47,53.13 IC3.6
  Top 0.254: IC3.39 55.22,59.53 53.2,61.55 47.53,61.55 47.46,61.61 R20.1 | IC1.44 44.14,29.03 43.81,29.36 | 25.61,58.09 25.84,58.09 26.17,58.09 27.75,59.66 30.49,59.66 LED1.C | C10.1 82.53,59.76 83.06,60.29 87.16,60.29 87.4,60.54 | C9.1 82.53,50.68 v82.53,49.71 | C8.1 82.41,35.38 82.94,35.91 87.9,35.91 X2.4 | C7.1 82.53,26.74 83.31,25.96 v84.26,25.96 | 30.46,59.62 LED1.C | LED2.C 30.42,59.57 LED1.C | 39.78,51.47 42.8,51.47 R11.2 | R7.1 41.46,53.21 39.92,51.68 39.84,51.59 | IC1.21 41.3,19.83 42.17,20.7 v42.54,20.7 42.8,20.7 44,21.92 44,22.5 | IC1.31 44,22.53 44,22.68 41.92,24.76 | IC1.62 37.8,39.16 | IC1.69 34.3,32.62 34.03,32.35 31.55,32.35 31.3,32.61 | 31.3,32.61 | v30.46,36.1 31.3,35.26 IC1.75 31.3,32.61 | IC1.84 31.4,28.03 v31.59,28.22 | IC1.100 v31.46,20.03 v31.47,20.03 | 75.38,11.72 75.38,11.71 v75.41,11.71
  Top 0.305: 64.42,61.17 65.05,60.54 65.17,60.54 65.18,60.53 IC3.24 67.18,60.54 67.88,60.54 v67.88,61.8 | IC3.27 64.44,62.66 64.45,61.19 64.42,61.17 | 64.42,61.17 64.42,59.85 v63.91,59.28 | v61.58,59.28 61.35,59.53 59.46,59.53 57.75,59.53 IC3.39 | v62.97,55.63 63.09,55.38 63.45,54.83 IC3.8 63.45,52.87 | v62.97,55.63 62.46,54.81 62.46,53.3 | 62.46,52.98 62.46,53.48 | 62.46,53.3 62.46,52.98 | 63.45,52.86 63.45,54.77 v62.97,55.63 | 59.95,52.88 59.95,53.38 59.95,53.63 59.95,56.65 v60.51,57.2 | 59.95,52.88 IC3.1 | 69.01,50.15 69.03,50.16 69.09,50.13 69.09,50.15 | 63.72,50.15 62.46,51.41 62.46,52.98 | 62.46,53.3 62.46,53.16 | 41.11,39.95 C15.2 40.76,39.5 42.74,39.5 43.81,38.43 43.81,30.87 | 43.81,30.87 43.81,29.36 | v31.47,20.03 31.21,20.03 | v41.92,31.25 41.92,24.76 | 43.81,30.87 v43.62,31.25 | v66.24,28.98 66.94,28.97 | C16.2 | 70.58,50.15 C3.1 | 68.76,50.02 68.89,50.15 | 37.8,39.16 v38.21,39.56 | 25.84,58.09 25.84,58.13 C1.- | 71.28,66.21 71.34,66.38 C19.- | 85.39,64.39 85.47,64.13 | 39.97,51.63 39.89,51.43 | 39.97,51.63 39.92,51.68 | 39.97,51.63 39.72,51.41
  Top 0.406: 39.72,51.47 39.84,51.59 40.57,52.32 v40.62,52.32 | IC2.34 66.94,28.97 59.3,28.97 58.43,28.16 57.04,28.16 57.03,28.17 | 57.03,28.17 56.98,28.22 | 57.03,28.17 IC2.12 | R19.1 76.81,14.6 75.38,13.17 75.38,11.72 77.27,11.72 | R14.1 76.79,19.68 v76.76,19.66 | v66.94,40.01 C16.2 | 63.72,50.15 68.89,50.15 69.09,50.15 70.58,50.15 | IC4.1 81.11,11.4 80.8,11.72 79.85,11.72 | 79.85,11.72 78.59,11.72 | 78.59,11.72 77.27,11.72 | IC4.2 79.84,11.71 79.85,11.72 | IC4.3 78.58,11.7 78.59,11.72 | IC4.4 77.3,11.68 77.27,11.72 | DEBUG.3 58.69,70.87 59.63,69.93 65.99,69.93 66.87,69.05 v66.87,67.09 | C15.2 40.66,40.95 41.55,41.83 44.74,41.83 46.19,43.28 47.72,44.79 | OSC1.2 62.04,43.58 | 64.16,40.04 C16.2 | C17.2 67.68,45.66 68.76,46.75 68.76,46.94 | 68.76,46.94 68.76,47.63 | 68.76,47.63 68.76,50.02 | 68.77,47.62 68.76,47.63 | C6.2 28.88,14.74 30.21,16.07 30.21,18.9 31.21,20.03 | C4.2 68.76,46.94 | 47.72,44.79 v47.59,44.92 | 47.72,44.79 49.67,44.79 50.3,44.16 52.05,44.16 C5.2 | v58.72,40.93 v56.43,40.93 | v62.81,13.57 v65.3,13.57 68.1,13.57 71.01,10.66 | 47.58,44.87 47.58,42.7 49.11,41.18 v49.11,41.2 v49.1,41.2 | 70.09,61.89 70.01,61.81 v67.89,61.81 v67.88,61.8
  Top 0.61: C13.2 85.47,67.78 83.19,69.99 83.19,73.08 82.12,74.09 80.05,74.09 IC5.1 | C13.2 85.47,64.13 85.47,62.48 87.4,60.54 X1.4 | v66.87,67.09 64.22,67.09 C12.2 | C14.2 71.59,10.09 v71,10.68 | OSC1.2 61.77,43.53 64.23,43.53 | C17.2 65.95,44.38 65.11,43.53 64.23,43.53 | 64.16,40.04 64.16,43.47 64.23,43.53 | C2.- 86.22,65.59 C13.2 | C19.- 68.83,66.65 68.45,67.03 66.94,67.03 | 71.28,66.53 71.28,66.21 72.29,65.2 77.83,65.2 78.65,64.39 85.39,64.39 85.46,64.45
  Top 0.813: 39.78,51.47 39.72,51.41 31.68,51.41 C1.- | 39.89,51.43 43.69,47.63 43.69,44.98 43.65,45.02 JTAG.6 | C11.2 95.5,43.37 v95.46,43.34 | 66.94,67.03 v66.87,67.09
  Top 1.016: v23.09,62.43 23.09,62.37 25.36,60.1 25.36,57.73 C1.-
  Bottom 0.254: v82.53,49.71 86.4,58.21 86.84,58.65 89.11,58.65 X1.4 | v84.26,25.96 85.33,25.96 86.21,26.84 86.21,33.64 86.97,34.4 88.99,34.4 X2.4
  Bottom 0.305: v61.58,59.28 v63.91,59.28 | v62.97,55.63 62.97,57.9 | 62.97,57.9 v61.58,59.28 | v60.51,57.2 60.51,58.21 v61.58,59.28 | 31.84,28.22 31.84,27.34 30.84,26.33 30.84,24.51 31.47,23.88 31.47,20.85 | 31.47,20.85 v31.47,20.03 | 31.84,28.22 31.84,31.25 28.32,34.78 28.32,35.66 28.76,36.1 v30.46,36.1 36.35,36.1 37.8,37.55 37.8,39.16 v38.21,39.56 44.95,39.56 47.72,42.34 47.72,44.79 v47.59,44.92 | 31.84,28.22 v31.59,28.22 | v43.62,31.25 v41.92,31.25 | v66.94,40.01 66.94,30.37 66.24,29.67 v66.24,28.98 | 32.03,3.14 32.03,18.21 33.73,19.91 33.73,20.41 33.29,20.85 31.47,20.85 | JTAG.6 43.47,45.13 43.75,44.98 | v67.88,61.8 67.88,66.09 v66.87,67.09 | C18.2 62.98,57.88 62.97,57.9
  Bottom 0.406: 89.09,34.51 88.94,34.51 | PL1.17 4.7,40 5.83,38.87 | 5.83,38.87 5.89,38.81 10.49,38.81 11.87,37.42 RN1.1 | PL1.26 6.82,29.94 5.51,31.25 5.51,38.56 5.83,38.87 | v76.76,19.66 76.76,14.55 76.73,14.52
  Bottom 0.61: RN4.1 5.43,61.59 4.22,60.38 PL1.1 PL1.3 | PL1.3 4.28,57.69 4.22,57.63 | PL1.3 4.28,55.32 4.22,55.26 4.24,55.24 PL1.5 PL1.7 | PL1.7 4.22,52.63 | 4.25,50.16 4.22,50.13 | 4.25,50.16 PL1.9 PL1.11 | PL1.7 4.28,50.19 4.25,50.16 | PL1.11 4.28,47.57 4.22,47.51 | PL1.13 4.28,44.94 4.22,44.88 | PL1.11 PL1.13 | PL1.13 4.28,42.69 4.22,42.63 4.28,42.57 PL1.15 4.28,40.07 4.22,40.01 4.22,40 PL1.17 | X3.4 89.2,19.77 91.59,17.38 91.59,16.75 85.63,10.79 v75.41,11.71 71.66,10.79 | 48.73,7 48.72,7 | 48.73,7 IDE.28 46.32,6.98 46.22,6.88 46.19,6.91 IDE.26 43.7,6.98 43.65,6.93 | 48.73,7 48.74,6.98 IDE.30 51.27,6.83 52.41,5.69 62.66,5.69 63.97,7 IDE.40 64.78,6.17 66.49,6.17 v71,10.68 | 43.65,6.93 43.59,6.88 | 43.65,6.93 IDE.24 41.2,6.98 41.11,6.89 | 41.11,6.89 IDE.22 | 41.11,6.89 38.66,4.44 IDE.19 38.57,4.41 38.59,4.38 37.41,3.14 32.03,3.14 14.71,3.14 13.97,3.88 13.97,5.13 15.71,6.87 IDE.2 | v47.59,44.92 43.81,44.92 43.75,44.98 | 71.66,10.79 71.11,10.79 v71,10.68 | v71,10.68 71.55,10.68 71.66,10.79
  Bottom 0.813: X3.4 89.2,19.86 89.22,19.88 89.34,19.75 93.59,19.75 96.97,23.13 96.97,31.25 93.61,34.61 X2.4 89.09,34.51 93.47,34.51 93.47,34.54 95.47,36.54 95.47,43.33 v95.46,43.34 95.41,43.39 95.41,55.5 92.16,58.76 89.32,58.76 89.24,58.84 89.2,58.8 X1.4 | 16.35,66.91 16.35,66.04 RN4.1
  Bottom 1.016: J1.3 17.04,74.29 17.04,72.45 17.1,72.45 18.55,71 | 18.55,71 23.46,71 24.54,72.07 24.54,74.21 24.6,74.28 J2.1 | 18.55,71 18.42,71 16.35,68.92 16.35,66.91 19.5,63.76 21.76,63.76 v23.09,62.43
  Bottom 1.27: J1.3 16.98,74.27 16.97,74.25 16.93,74.29 J1.2
  other vias: 68.77,46.95 70.07,61.89
  pour Bottom (isolate 0.254): 0.09,80.03 99.89,80.03 99.89,0.06 0,0.06 0,80.03
IDE8
  Top 0.254: IDE.4 19.2,6.98 21.85,9.63 26.53,9.63 31.3,14.41 IC1.1 31.3,17.93
IDE9
  Top 0.254: IDE.6 20.79,7.2 22.47,8.88 26.78,8.88 33.8,15.9 IC1.6
IDE10
  Top 0.254: IDE.8 24.47,8.13 26.97,8.13 34.8,15.96 IC1.8
IDE11
  Top 0.254: 35.31,17.95 IC1.9 35.3,15.61 26.7,7.02 25.91,7.02 IDE.10
IDE12
  Top 0.254: IDE.12 28.41,7.82 35.8,15.21 IC1.10
IDE13
  Top 0.254: IDE.14 30.95,9.3 | 30.95,9.3 30.95,9.36 | IC1.11 36.3,14.65 30.95,9.3
IDE14
  Top 0.254: IDE.16 33.49,10.72 | 33.49,10.72 33.49,10.77 | IC1.12 36.8,14.03 33.49,10.72
IDE15
  Top 0.254: IDE.18 36.03,12.18 37.3,13.45 IC1.13
MHZ1  (via drill 0.3, 0.5)
  Top 0.254: v42.37,15.62 42.37,16.25 41.8,16.82 41.8,17.32 IC1.22 | v29.83,34.71 25.17,39.38 v25.17,40.89 | v8.85,46.94 8.85,50.21 7.84,51.22 7.84,56.45 7.15,57.14 PL1.4
  Bottom 0.254: v42.37,15.62 40.79,15.62 31.59,24.76 31.59,25.96 32.47,26.84 32.47,32.07 v29.83,34.71 | v25.17,40.89 21.01,40.89 16.85,45.05 10.74,45.05 v8.85,46.94
N$1
  Bottom 0.61: IDE.20 38.59,6.98 38.59,12.06 JP1.2
N$2
  Top 1.27: J1.4 19.52,76.08 18.3,77.3 10.49,77.3 9.54,76.36 9.54,69.74 10.97,68.31 | 10.97,68.31 11.05,68.23 | F1.+ 10.97,68.31
N$3  (via drill 0.3)
  Top 0.254: IC1.48 48.57,31.03 v48.92,30.68 | v51.44,30.93 51.44,32 50.81,32.63 47.72,32.63 44.7,35.66 44.7,38.68 v42.37,41.01
  Bottom 0.254: v48.92,30.68 51.19,30.68 v51.44,30.93 | JTAG.2 33.49,44.93 33.48,44.92 37.39,41.01 v42.37,41.01
N$4  (via drill 0.3)
  Top 0.254: IC1.47 47.3,30.53 v47.78,30.05 | v52.7,30.93 52.7,31.81 52.13,32.38 51.31,33.14 48.1,33.14 45.26,35.97 45.26,39.5 v43.75,41.01
  Bottom 0.254: v47.78,30.05 48.16,30.05 48.41,29.8 51.5,29.8 52.63,30.93 v52.7,30.93 | v43.75,41.01 43.75,41.08 42.87,41.96 38.14,41.96 36,44.1 36,44.92 36.03,44.95 JTAG.3
N$5  (via drill 0.3)
  Top 0.254: IC1.83 26.92,28.53 v26.61,28.22
  Bottom 0.254: v26.61,28.22 26.61,35.15 28.63,37.17 31.15,37.17 32.22,38.24 32.22,46.62 32.91,47.31 37.64,47.31 38.59,46.37 38.59,44.98 38.57,45 JTAG.4
N$6  (via drill 0.3)
  Top 0.254: IC1.45 46.85,29.53 47.47,28.92 v48.79,28.92 | v52.19,28.98 53.89,30.68 53.89,31.31 53.58,31.63 53.58,32 51.88,33.71 48.35,33.71 45.96,36.1 45.96,40.07 v45.01,41.01
  Bottom 0.254: v48.79,28.92 52.07,28.92 52.13,28.98 v52.19,28.98 | v45.01,41.01 44.76,41.33 43.31,42.9 41.67,42.9 41.1,43.47 41.1,44.92 41.11,44.92 JTAG.5
N$7
  Top 0.406: R21.1 39.6,64.13 37.7,66.02 37.7,68.73 35.5,70.94 35.06,70.94 34.74,71.25 34.74,74.34 34.76,74.32 J2.5
N$8
  Top 0.254: IC3.4 61.45,52.48 61.83,52.1 61.83,48.51 OSC1.3
N$9
  Top 0.254: LED2.A R23.2
N$10
  Top 0: IC3.7 62.95,53.62 62.94,53.63
  Top 0.254: 62.94,53.63 62.94,51.7 63.72,50.9 68.64,50.9 69.33,51.6 73.05,51.6 73.61,51.03 73.61,49.89 C3.2 75.66,49.85 R5.2
N$11
  Top 0.254: C4.1 75.71,46.94 R5.1
N$12  (via drill 0.5)
  Top 0.254: R6.1 74.68,55.84 74.68,54.68 v74.24,54.24 73.97,53.97 66.39,53.97 65.61,54.75 64.45,54.75 64.45,52.85 64.45,52.86 IC3.10
  Bottom 0.254: DEBUG.5 62.69,70.84 63.6,69.93 69.14,69.93 72.61,66.46 72.61,58.65 73.42,57.83 73.42,55.06 v74.24,54.24
N$13
  Top 0.406: R10.1 39.45,66.67 38.52,67.6 38.52,71.25 39.78,72.51 39.78,74.34 J2.7
N$14
  Top 0.254: IC3.26 64.95,61.86 64.95,63.16 65.11,63.32 75.82,63.32 76.95,62.18 76.95,53.36 79.28,51.03 79.28,31 80.23,30.05 82.5,30.05 R4.1
N$15
  Top 0.406: R20.2 39.81,61.59 36.88,64.51 36.88,68.29 35.31,69.87 31.34,69.87 29.64,71.57 29.64,74.21 29.7,74.28 J2.3
N$16  (via drill 0.5)
  Top 0.254: IC3.25 65.45,61.88 65.45,62.81 65.55,62.81 75.57,62.81 76.39,61.99 76.39,53.17 78.4,51.16 v78.4,32.19 | v80.73,32.19 R3.1
  Bottom 0.254: v78.4,32.19 v80.73,32.19
N$17
  Top 0.813: D2.C 25.74,65.4 28.22,67.88 34.72,67.88 34.78,67.94 | 34.78,67.94 34.84,68 | 34.78,67.94 D1.A
N$18
  Top 0.813: D1.C 25.03,67.94 27.09,70 27.09,74.25 J2.2
N$19  (via drill 0.5)
  Top 0.254: IC3.29 63.45,62.26 63.45,61.86 63.45,63.88 64.1,64.51 76.32,64.51 80.98,59.85 v80.98,59.03 | v80.98,54.75 81.76,53.97 R2.1
  Bottom 0.254: v80.98,59.03 v80.98,54.75
N$20
  Top 0.254: IC3.28 63.95,61.85 63.95,63.67 64.16,63.88 76.13,63.88 79.91,60.1 79.91,57.46 80.86,56.51 R1.1
N$21
  Top 0.254: X2.2 89.18,30.09 R4.2 84.28,30.05 C7.2 85.12,27.99 85.52,27.59 85.52,18.96 X3.2
N$22
  Top 0.254: C8.2 84.16,32.27 R3.2 89.12,32.19 X2.3 91.02,32.11 91.63,31.5 91.63,29.67 90.81,28.85 87.66,28.85 86.65,27.85 86.65,24.51 91,20.16 91,19.09 X3.3
N$23
  Top 0.254: X1.2 88.93,53.97 R2.2 84.24,51.85 C9.2
N$24
  Top 0.254: X1.3 88.93,56.51 R1.2 84.28,56.55 C10.2
N$25
  Top 0.406: R9.1 39.94,69.21 39.72,69.43 39.72,70.43 40.73,71.44 44,71.44 44.88,72.32 44.88,74.25 J2.9 44.94,74.29 44.95,74.28
N$26  (via drill 0.5)
  Top 0.254: IC3.16 66.78,56.53 68.43,56.53 v69.01,55.94 | v47.47,66.63 45.47,66.63 R10.2
  Bottom 0.254: v69.01,55.94 69.01,67.41 67.88,68.54 49.36,68.54 47.47,66.65 | 47.47,66.65 47.46,66.66 | v47.47,66.63 47.47,66.65
N$28
  Top 0: IC3.47 58.22,55.51 58.22,55.53
  Top 0.254: 58.63,55.53 58.22,55.53 55.18,55.53 53.64,53.99 49.11,53.99 48.29,53.17 44.54,53.17 R7.2 | 58.63,55.53 IC3.47
N$29  (via drill 0.5)
  Top 0.254: IC3.18 66.77,57.53 66.76,57.53 70.28,57.53 71.6,58.84 71.6,61.8 v71.53,61.87 | v47.47,69.13 45.47,69.13 R9.2
  Bottom 0.254: v71.53,61.87 71.53,66.53 68.83,69.24 47.47,69.24 | 47.41,69.24 47.47,69.24 | v47.47,69.13 47.47,69.24
N$30
  Bottom 0.813: 91.95,19.84 91.95,22.81
N$31  (via drill 0.5)
  Top 0.406: R13.2 82.98,22.22 v83,22.24
  Bottom 0.406: v83,22.24 84.75,22.24 X3.1
N$32
  Bottom 0.813: 91.88,36.16 91.88,34.59
N$33
  Bottom 0.813: 90.69,13.8 89.87,14.62
N$34
  Bottom 0.813: 93.58,48.51 95.35,48.51
N$35
  Bottom 0.813: 91.88,58.84 91.88,60.23
N$36
  Top 0: IC3.48 58.22,55.01 58.22,55.03
  Top 0.254: 58.65,55.03 58.22,55.03 55.44,55.03 53.7,53.3 49.3,53.3 48.22,52.23 46.27,52.23 45.45,51.41 44.52,51.41 R11.1 | 58.65,55.03 IC3.48
N$37
  Top 0.254: LED1.A 34.83,59.65 R22.2
N$38  (via drill 0.5)
  other vias: 63.97,11.84
N$41  (via drill 2.4 pad 4.2)
  other vias: 91.95,24.51
N$43  (via drill 0.5)
  Top 0.254: IC3.11 64.95,52.64 65.61,51.98 68.26,51.98 68.95,52.67 74.81,52.67 75.82,53.68 75.82,58.72 v75.12,59.41
  Bottom 0.254: v75.12,59.41 75.12,59.47 73.3,61.3 73.3,67.16 67.19,73.27 55.22,73.27 54.59,72.64 54.59,71.47 DEBUG.1
N$50  (via drill 0.5)
  Top 0.254: IC3.3 60.95,52.1 60.51,51.66 58.05,51.66 57.8,51.91 56.32,51.91 R24.2 55.19,51.94 v54.9,51.66 | C5.1 52.07,49.01 52.57,49.52 v53.64,49.52
  Bottom 0.254: v53.64,49.52 53.64,50.4 v54.9,51.66
N$51  (via drill 2.4 pad 4.2)
  other vias: 91.95,61.87
N$52  (via drill 2.4 pad 4.2)
  other vias: 91.95,48.64
N$53  (via drill 2.4 pad 4.2)
  other vias: 91.95,37.67
N$54  (via drill 2.4 pad 4.2)
  other vias: 91.95,12.54
RD#  (via drill 0.5)
  Top 0: IC3.43 58.22,57.51 58.22,57.53
  Top 0.254: 58.63,57.53 58.22,57.53 52.43,57.53 50.29,57.53 v49.17,58.65 | 58.63,57.53 IC3.43 | v34.74,49.33 34.74,42.34 35.31,41.77 35.3,41.76 IC1.67
  Bottom 0.254: v34.74,49.33 34.74,50.72 35.3,51.27 36.7,51.27 43.14,57.71 48.22,57.71 v49.17,58.65
RDY  (via drill 0.5)
  Top 0.254: v12.5,14.11 14.86,14.11 R16.2
  Bottom 0.254: IDE.27 48.73,4.29 47.72,3.28 40.16,3.28 38.71,1.83 13.95,1.83 12.5,3.28 v12.5,14.11
RNW
  Top 0.254: PL1.2 17.07,60.32 19.12,58.28 19.12,56.45 22.9,52.67 22.9,49.96 27.43,45.42 27.43,42.27 33.3,36.41 IC1.71 33.3,33.96 33.29,33.96
RXF#  (via drill 0.5)
  Top 0: IC3.41 58.22,58.51 58.22,58.53
  Top 0.254: 58.65,58.53 58.22,58.53 54.65,58.53 53.83,58.53 v52.95,59.41 | 58.65,58.53 IC3.41 | v37.45,48.45 37.32,48.32 37.32,43.41 35.8,41.88 IC1.66
  Bottom 0.254: v37.45,48.45 38.65,49.64 47.03,49.64 48.48,51.09 48.48,56.57 51.31,59.41 v52.95,59.41
SCL  (via drill 0.5)
  Top 0.254: v45.89,14.74 43.31,17.32 IC1.25 | v61.01,10.21 61.01,9.32 62.71,7.62 62.71,3.46 64.67,1.45 77.9,1.45 78.59,2.14 78.59,4.37 IC4.6
  Bottom 0.254: v45.89,14.74 56.48,14.74 v61.01,10.21
SDA  (via drill 0.3, 0.5)
  Top 0.254: v61.48,14.55 73.11,14.55 | 73.11,14.55 75.69,17.14 R18.1 | 73.11,14.55 73.11,9.83 75.38,7.56 76.01,7.56 77.33,6.24 77.33,4.41 IC4.5 | IC1.20 40.8,16.75 v41.1,16.44
  Bottom 0.254: v41.1,16.44 59.61,16.44 v61.48,14.55
SWP
  Top 0.254: 87.64,5.71 84.97,8.38 | 84.97,8.38 84.97,12.88 83.22,14.63 80.09,14.63 R19.2 | 84.97,8.38 84.97,8.21 83.88,7.12 80.92,7.12 79.85,6.05 IC4.7
  Top 0.406: IC4.7
  Top 0.61: JP3.1 87.64,5.71
TXE#  (via drill 0.5)
  Top 0: IC3.42 58.22,58.01 58.22,58.03
  Top 0.254: 58.65,58.03 58.22,58.03 53.63,58.03 52.44,58.03 v52,58.46 | 58.65,58.03 IC3.42 | v39.72,48.07 39.72,43.6 36.8,40.68 IC1.64
  Bottom 0.254: v39.72,48.07 40.54,48.89 47.28,48.89 49.3,50.9 49.3,56.39 51.37,58.46 v52,58.46
UBVCC  (via drill 0.5)
  Top 0.254: IC3.19 69.37,58.03 v70.59,59.26 | v76.51,22.24 78.34,22.24 R13.1
  Top 0.305: R13.1 78.36,21.46 78.84,20.98 79.47,20.98 80.04,20.41 80.04,19.7
  Top 0.406: 80.04,19.7 R14.2
  Bottom 0.254: v70.59,59.26 72.3,57.54 72.35,56.89 72.35,54.75 74.94,52.16 77.77,52.16 78.72,51.22 78.72,33.89 76.51,31.69 v76.51,22.24
VCC  (via drill 0.3, 0.5, 0.6)
  Top 0: 32.78,18.03 IC1.4
  Top 0.254: R16.1 16.59,14.11 17.35,14.11 17.98,14.74 17.98,17.46 20.73,20.2 22.69,20.2 v22.71,20.22 23.52,21.03 IC1.98 | JTAG.1 30.95,39.51 33.8,36.66 IC1.70 | R22.1 36.55,62.27 34.74,64.07 34.74,65.38 D2.A | IC1.3 32.3,19.31 | 32.3,19.31 32.3,20.43 31.7,21.04 31.68,21.02 29.42,21.02 | IC1.4 32.8,19.23 | 32.8,19.23 32.8,19.33 | 32.8,19.33 32.79,19.34 32.33,19.34 32.3,19.31 | v32.84,16.11 33.3,16.58 IC1.5 33.3,19.31 33.28,19.33 32.8,19.33 | 32.78,19.32 32.78,19.25 32.8,19.23 | v44,15.06 43.48,15.58 43.48,15.85 42.3,17.02 IC1.23 42.3,19.06 43.27,20.03 IC1.26 | IC1.38 43.99,26.03 42.81,27.22 | IC1.51 43.3,32.55 42.84,32.09 42.81,32.06 | 42.3,32.51 IC1.53 42.3,36.29 42.31,36.3 42.05,36.56 41.45,36.56 41.44,36.57 | IC1.54 41.8,32.56 41.85,32.51 | IC1.55 41.3,32.53 41.32,32.51 | IC1.56 40.8,32.54 40.77,32.51 | IC1.57 40.3,32.53 40.32,32.51 | IC1.58 39.8,32.51 | IC1.59 39.3,32.51 | 38.8,33.92 IC1.60 38.8,36.05 39.32,36.57 39.94,36.57 39.96,36.58 40.03,36.58 40.35,36.27 | 38.8,33.92 38.8,32.52 38.81,32.51 | IC1.65 36.3,32.52 36.31,32.51 | 38.8,34.57 38.81,34.57 38.81,33.93 38.8,33.92 | IC1.88 24.97,26.03 v22.71,28.29 | v64.04,12.03 61.59,12.03 61.47,11.91
  Top 0.305: 42.81,32.06 42.81,27.22 | IC2.40 67.75,33.77 65.49,33.77 61.14,38.12 61.14,39.94 C16.1 | v25.04,38.05 31.4,31.69 34.49,31.69 35.31,32.51 36.31,32.51 38.81,32.51 39.3,32.51 39.8,32.51 40.32,32.51 40.77,32.51 41.32,32.51 41.85,32.51 42.3,32.51 42.43,32.51 42.84,32.09 | C1.+ 21.34,57.76 21.39,57.76 | C14.1 71.59,5.5 C14.1
  Top 0.406: 32.22,77.25 32.22,77.24 | 37.26,77.25 37.26,77.24 37.3,77.2 J2.6 | IC2.11 57.98,28.97 59.25,30.24 v59.56,30.24 59.56,32.51 59.31,32.76 59.31,39.5 59.75,39.94 61.14,39.94 C16.1 | IC2.33 68.38,28.17 68.38,28.16 60.76,28.16 60.32,27.72 v59.56,27.72 | IC4.8 81.11,2.83 81.49,2.46 88.67,2.46 90.5,4.28 90.5,7.81 90.06,8.25 JP3.2 | 40.29,36.21 40.35,36.27 C15.1 | C6.1 v23.15,14.74
  Top 0.61: JP3.2 87.97,8.38 87.72,8.38 86.47,9.63 86.47,13.63 84.47,15.63 | 83.02,17.08 82.97,17.13 82.98,17.14 R18.2 83.02,17.08 | 84.47,15.63 83.02,17.08 | 84.47,15.63 90.47,15.63 91.72,16.88 95.85,21.11 97.17,22.36 97.17,68.17 93.9,71.44 92.58,71.44 91.25,72.77 91.25,73.96 87.85,77.36 75.31,77.36 75.25,77.3 | 19.52,61.61 19.5,61.61 19.47,61.59 RN3.1 | C14.1 69.33,5.48 68.57,6.24 68.57,9.83 66.43,11.97 64.1,11.97 64.04,11.91 61.47,11.91 61.16,11.91 R17.2 | v74.37,5.48 C14.1 71.47,5.48
  Top 0.813: 19.52,61.61 19.52,61.58 | 32.22,77.24 J2.4 | JTAG.1 30.95,44.93 30.96,44.92 31.02,44.98 31.02,47 30.96,47 21.39,56.57 | F1.- 20.46,68.33 20.44,68.35 22.27,70.18 22.27,76.04 23.48,77.25 32.22,77.25 37.26,77.25 37.37,77.3 75.25,77.3 L1.2
  Top 1.016: F1.- 20.46,68.25 20.44,62.56 19.5,61.61 | 19.52,61.58 19.52,61.53 21.39,59.66 21.39,57.76 21.39,56.57
  Bottom 0.305: 44,12.06 v44,15.06 | v59.56,30.24 60,30.43 62.27,30.43 63.41,31.56 65.17,31.56 65.67,31.06 65.67,30.11 64.98,29.42 64.98,21.51 63.97,20.5 63.97,12.1 v64.04,12.03 | v32.84,16.11 37.21,16.12 40.35,12.88 JP1.1 | 22.65,28.38 22.72,28.38 v22.71,28.29 | v23.15,14.74 23.15,15.06 | JP3.2 88.22,8.26 88.04,8.25
  Bottom 0.406: v59.56,30.24 v59.56,27.72 | v22.71,28.29 v22.71,20.22 23.17,19.67 23.17,16.7 23.15,15.06 | JTAG.1 30.95,44.15 25.1,38.3 v25.04,38.05 25.04,38.24 24.28,37.48 22.77,37.48 22.77,28.41 22.65,28.29 22.65,28.38 22.65,37.42 22.58,37.48 15.65,37.48 15.68,37.46 RN2.1 | 34.74,65.39 34.75,65.4 D2.A
  Bottom 0.61: JP1.1 44,12.06 44.04,12.06 47.09,9.01 63.47,9.01 64.04,9.58 v64.04,12.03 63.97,12.1 63.97,12.09 | 88.04,8.25 77.14,8.25 v74.37,5.48
  Bottom 0.813: J2.4 32.22,66.72 32.85,66.09 34.05,66.09 34.74,65.39
VCC3V3  (via drill 0.5, 0.6)
  Top 0: IC3.40 58.22,59.01 58.22,59.03
  Top 0.254: 74.68,57.58 R6.2 | 60.45,54.75 IC3.2 60.45,52.36 60.32,52.23 59.25,52.23 58.87,52.61 58.87,53.23 58.49,53.61 56.32,53.61 R24.1 | 67,57.03 62.36,57.03 62.16,57.23 | R23.1 41.04,57.52 41.23,57.71 | 41.23,57.39 41.23,56.51 | 41.23,56.51 41.23,55.25 41.61,54.87 R25.1 | R8.1 41.23,56.51
  Top 0.305: C12.1 60.62,66.67 62.95,64.32 62.95,62.18 62.95,62.2 IC3.30 62.95,58.48 62.16,57.23 62.06,57.07 | 62.02,57.02 62.06,57.07 | 62.15,57.03 62.1,57.03 60.95,55.88 60.84,55.63 | 62.15,57.03 IC3.17 72.87,57.03 73.42,57.58 | 60.84,55.63 60.45,54.75 | 62.15,57.03 62.15,57.02 62,57.16 | 57.82,59.03 58.22,59.03 60.13,59.03 62,57.16 | 57.82,59.03 IC3.40 | IC5.4 85.97,72.13 85.96,72.07 | 73.42,57.58 74.68,57.58 | v75,61.43 73.3,59.72 73.3,57.71 73.42,57.58 | 41.23,57.39 41.23,57.71 41.23,59.03 | 41.23,59.03 v41.23,60.29 | R12.2 41.25,58.17 41.23,59.03 | 60.84,55.63 v60.95,55.63 | 62.06,57.07 61.97,57.13 62,57.16
  Top 0.406: OSC1.4 56.65,49.12 57.11,49.58 v59.38,49.58
  Top 0.61: IC5.4 86.08,72.13 | 85.96,72.13 85.97,72.13 | C13.1 80.54,66.35 v80.23,66.67 | 56.36,47.49 OSC1.4 | C17.1 64.44,48.66 v63.97,48.64 | C2.+ 88.36,68.8 87.47,69.68 | 87.47,69.68 85.96,71.19 | v86.34,68.86 86.65,68.86 87.47,69.68
  Top 0.813: 85.96,71.19 85.96,72.13
  Bottom 0.254: 79.22,66.66 81.52,66.67
  Bottom 0.305: v41.23,60.29 41.23,61.49 42.18,62.43 42.18,74.09 J2.8 | C18.1 64.51,55.46 62.84,53.79
  Bottom 0.406: v60.95,55.63 62.84,53.79 63.41,53.23 63.97,53.23 64.98,52.23 64.98,51.35 63.97,50.33 63.97,48.7 | 63.97,48.7 63.09,49.58 v59.38,49.58 | 63.97,48.7 v63.97,48.64
  Bottom 0.61: v86.34,68.86 84.65,66.73 81.52,66.67 v80.23,66.67 79.14,66.67 71.52,74.29 71.52,74.33 70.38,75.48 47.46,75.48 | J2.10 47.46,75.48 | 47.46,75.48 47.43,75.51 46.33,76.61 43.44,76.61 42.37,75.54 42.37,74.3 J2.8 | 79.22,66.66 76.08,66.66 74.87,65.46 74.87,61.55 v75,61.43
VCC_RF
  Top 0.406: L1.1 65.48,72.16 DEBUG.6
  Top 0.61: 76.04,71.98 76.7,71.32 78.47,69.55 79.11,69.54 78.46,68.89 78.46,67.47 77.64,66.65 C19.+
  Top 0.813: L1.1 75.88,72.13 76.04,71.98 77.77,73.71 77.77,75.54 78.28,76.04 87.22,76.04 89.68,73.58 89.68,72.58 92.2,70.06 93.33,70.06 95.79,67.6 95.79,57.33 90.2,51.74 X1.1 89.2,51.5 87.91,50.21 87.91,44.24 C11.1 88.78,41.91 89.49,41.2 93.33,41.2 95.28,39.25 95.28,31.31 91.69,27.72 89.31,27.72 X2.1 | 79.11,69.54 IC5.3
WR  (via drill 0.5)
  Top 0: IC3.44 58.22,57.01 58.22,57.03
  Top 0.254: IC3.44 58.65,57.03 58.22,57.03 51.23,57.03 49.47,57.03 v47.34,59.16 | v32.1,49.39 32.1,43.47 34.8,40.76 34.8,34.08 IC1.68
  Bottom 0.254: v47.34,59.16 47.28,59.22 47.28,59.12 46.39,58.23 42.9,58.23 36.51,51.84 34.54,51.84 v32.1,49.39

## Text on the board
tNames: RetroClinic | DataCentre | Iss.3 | Ver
